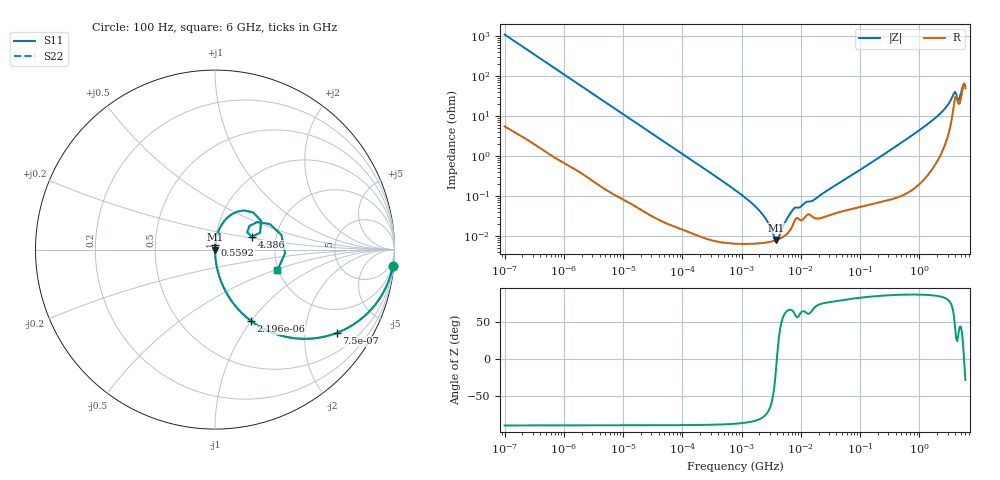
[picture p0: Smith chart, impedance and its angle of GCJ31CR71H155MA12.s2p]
!Murata Part Number: GCJ31CR71H155MA12
!These Parameters are Measured in Series Mode Connection
!Data Generated on Mar 13, 2026
!  o--ll--o
!Port1  Port2
!  o------o
!Operation Temp=25[degC], DC Bias Voltage=0[V]
!Freq. Start=100[Hz] Stop=6[GHz] 401[Steps]
# Hz S RI R 50
!Freq.(Hz) S11(Real) S11(Imag) S21(Real) S21(Imag) S12(Real) S12(Imag) S22(Real) S22(Imag)
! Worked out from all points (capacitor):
!   401 points, 100 Hz to 6 GHz, reference 50 ohm
!   read as one part in series: C = 1.46 uF near 109 Hz
!   lowest |Z| = 7.88 mohm at 3.882 MHz (marker M1)
!   series resonance near 3.942 MHz, so ESL is about 1.1 nH
!   S11 on the Smith chart (normalised r, x): 100 Hz: 1, -22; 750 Hz: 1.02, -2.92; 2.196 kHz: 1.01, -1.00; 559.2 MHz: 1.00, +0.05; 4.386 GHz: 1.50, +0.23; 6 GHz: 1.98, -0.52
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100  0.9912 -0.0911  0.00883 0.0911  0.00883 0.0911  0.9912 -0.0911
335  0.9128 -0.2793  0.0872 0.2793  0.0872 0.2793  0.9128 -0.2793
750  0.68 -0.4636  0.32 0.4636  0.32 0.4636  0.68 -0.4636
1227  0.4448 -0.4938  0.5552 0.4938  0.5552 0.4938  0.4448 -0.4938
2008  0.2323 -0.419  0.7677 0.419  0.7677 0.419  0.2323 -0.419
2196  0.2023 -0.3984  0.7977 0.3984  0.7977 0.3984  0.2023 -0.3984
5882  0.0352 -0.181  0.9648 0.181  0.9648 0.181  0.0352 -0.181
40335  0.00101 -0.0276  0.999 0.0276  0.999 0.0276  0.00101 -0.0276
774597  6.55e-05 -0.0014  0.9999 0.0014  0.9999 0.0014  6.55e-05 -0.0014
1983483  6.49e-05 -0.000426  0.9999 0.000426  0.9999 0.000426  6.49e-05 -0.000426
3882480  7.83e-05 -8.7e-06  0.9999 8.7e-06  0.9999 8.7e-06  7.83e-05 -8.7e-06
4440638  8.49e-05 7.01e-05  0.9999 -7.01e-05  0.9999 -7.01e-05  8.49e-05 7.01e-05
7599586  0.000211 0.000424  0.9998 -0.000424  0.9998 -0.000424  0.000211 0.000424
1.555665e7  0.000302 0.000682  0.9997 -0.000682  0.9997 -0.000682  0.000302 0.000682
3.124326e8  0.000968 0.0134  0.999 -0.0134  0.999 -0.0134  0.000968 0.0134
5.59173e8  0.00165 0.0239  0.9984 -0.0239  0.9984 -0.0239  0.00165 0.0239
1.95892e9  0.0154 0.0921  0.9846 -0.0921  0.9846 -0.0921  0.0154 0.0921
2.931063e9  0.0528 0.1607  0.9472 -0.1607  0.9472 -0.1607  0.0528 0.1607
3.666503e9  0.1624 0.2183  0.8376 -0.2183  0.8376 -0.2183  0.1624 0.2183
4.385646e9  0.2052 0.0719  0.7948 -0.0719  0.7948 -0.0719  0.2052 0.0719
5.245841e9  0.3049 0.1425  0.6951 -0.1425  0.6951 -0.1425  0.3049 0.1425
6e9  0.3478 -0.1143  0.6522 0.1143  0.6522 0.1143  0.3478 -0.1143
